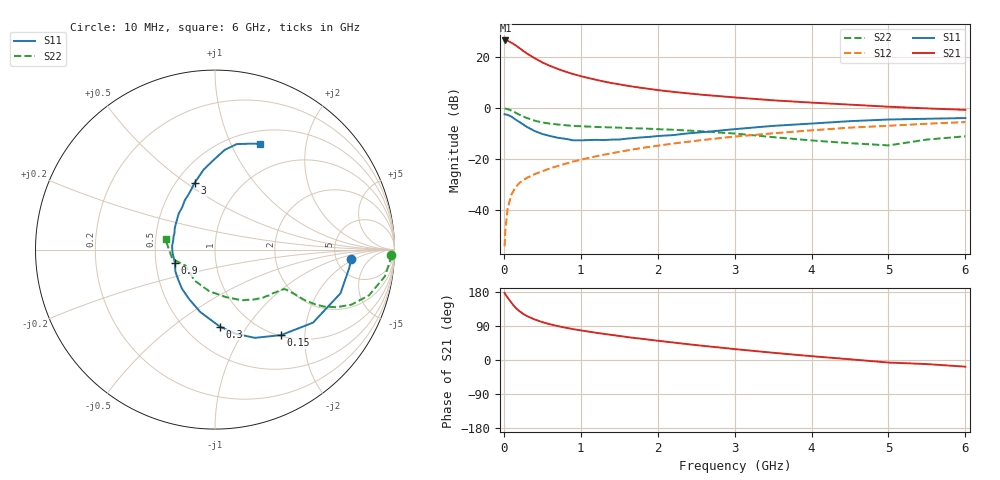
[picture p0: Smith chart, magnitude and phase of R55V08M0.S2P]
! SIEMENS Small Signal Semiconductors
! BFR183
! Si NPN RF Bipolar Junction Transistor in SOT23
! VCE = 5 V  IC = 8 mA
! Common Emitter S-Parameters:  May  1996
# GHz  S  MA  R  50
!  f  S11  S21  S12  S22
! GHz  MAG  ANG  MAG  ANG  MAG  ANG  MAG  ANG
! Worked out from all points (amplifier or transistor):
!   36 points, 10 MHz to 6 GHz, reference 50 ohm
!   highest |S21| = 26.5 dB at 20 MHz (marker M1)
!   |S21| within 3 dB of that: start of sweep to 204.1 MHz
!   unconditionally stable (mu >= 1): 866.1 MHz to 2.626 GHz
!   at 250 MHz: K = 0.55, MSG = 25.3 dB, |S12| = -28.2 dB
!   at 1.4 GHz: K = 1.06, MAG = 12.3 dB, |S12| = -17.6 dB
!   at 6 GHz: K = 0.88, MSG = 2.4 dB, |S12| = -5.4 dB
!   lowest NFmin = 1.30 dB at 450 MHz
!   S11 on the Smith chart (normalised r, x): 10 MHz: 6.91, -1.74; 150 MHz: 1.02, -1.52; 300 MHz: 0.72, -0.76; 900 MHz: 0.63, -0.10; 3 GHz: 0.62, +0.54; 6 GHz: 0.65, +1.30
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0.01  0.7606 -4.0  21.04 176.8  0.002 90.9  0.9834 -1.8
0.02  0.7549 -7.8  21.1 173.4  0.0042 85.6  0.9779 -3.6
0.05  0.7404 -19.2  20.78 164.4  0.0109 79.7  0.9576 -9.0
0.1  0.6811 -36.7  19.02 150.9  0.0207 73.5  0.8956 -16.5
0.15  0.6017 -52.4  17.07 138.4  0.0279 66.9  0.8197 -22.0
0.2  0.5394 -65.7  15.1 129.3  0.0342 64.6  0.7477 -25.4
0.25  0.4818 -76.4  13.23 122.0  0.0391 62.3  0.6879 -27.5
0.3  0.4298 -86.4  11.75 115.9  0.0434 61.7  0.6414 -28.6
0.4  0.3578 -103.1  9.516 107.1  0.0512 60.9  0.5698 -29.4
0.5  0.3128 -116.9  7.849 99.9  0.0583 61.2  0.5252 -29.3
0.6  0.2857 -129.9  6.714 94.4  0.0663 61.7  0.4983 -29.2
0.7  0.264 -141.3  5.871 89.5  0.0739 62.6  0.4794 -29.2
0.9  0.2355 -161.2  4.656 81.5  0.0902 63.5  0.4502 -29.4
1.1  0.2377 -176.8  3.887 75.0  0.1063 63.6  0.4361 -30.9
1.3  0.2379 168.4  3.321 69.0  0.123 63.0  0.4242 -32.4
1.6  0.2537 152.1  2.749 60.7  0.1487 62.0  0.4085 -36.0
2.2  0.2976 128.0  2.085 46.2  0.203 58.1  0.3784 -45.0
3  0.3886 107.0  1.623 28.8  0.2781 50.2  0.3195 -62.1
3.5  0.4506 98.0  1.425 19.1  0.3222 44.3  0.2715 -77.1
4.5  0.5574 84.5  1.172 1.9  0.4164 32.3  0.2069 -123.3
5.5  0.6204 72.0  0.989 -10.8  0.496 20.4  0.2435 -167.6
6  0.6407 67.0  0.928 -17.6  0.5343 12.6  0.2815 168.4
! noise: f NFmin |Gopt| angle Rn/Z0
0.45  1.3  0.17  43  0.21
0.9  1.35  0.21  115  0.2
1.8  2.05  0.33  -177  0.14
